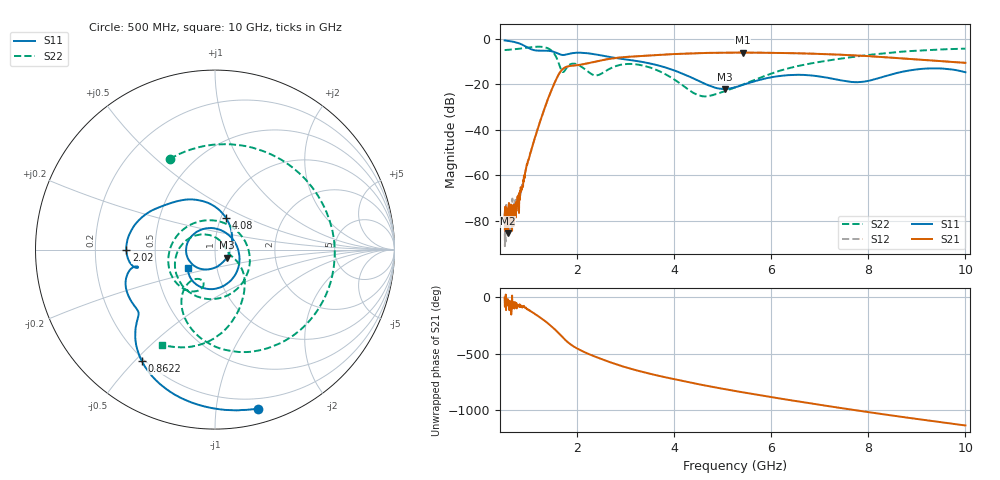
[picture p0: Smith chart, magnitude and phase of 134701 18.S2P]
!  2-Port S-parameters saved by WinCal
! VAR MeasName=S-Parameters (CALIBRATED_DATA) read from VNA (N5242A)
! VAR MeasDate=2013-7-3 16:31:00
! VAR NAME=134701 18
! VAR FILENAME=134701 18.S2P
! VAR DATE=2013-7-3 16:31:00
! VAR PHYS_PORTS=1,2
# Hz S MA R 50
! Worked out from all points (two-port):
!   1601 points, 500 MHz to 10 GHz, reference 50 ohm
!   highest |S21| = -6.09 dB at 5.41 GHz (marker M1); lowest = -85.5 dB at 565.3 MHz (marker M2)
!   |S21| within 3 dB of the highest: 2.592 GHz to 8.999 GHz (6.407 GHz wide, 111 % of centre)
!   lowest |S11| = -22.1 dB at 5.036 GHz (marker M3), VSWR 1.17, Z = 56.6 - j5.16 ohm
!   |S11| at or under -10 dB: 3.286 GHz to end of sweep
!   |S22| runs from -25.4 to -3.5 dB; largest |S21 - S12| = 0.0022
!   S11 on the Smith chart (normalised r, x): 500 MHz: 0.12, -1.30; 862.2 MHz: 0.19, -0.52; 2.02 GHz: 0.34, -0.00; 4.08 GHz: 1.06, +0.39; 10 GHz: 0.72, -0.15
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5e8  0.9175 -74.8  0.0001227 -4.8  0.000148 -52.6  0.5644 116.6
5.653125e8  0.8996 -83.9  5.304e-05 -55.7  0.0001652 -62.7  0.5707 107.3
7.196875e8  0.8404 -105.2  0.0002006 -45.6  0.0002437 -47.8  0.5909 83.7
8.621875e8  0.7426 -123.3  0.0005362 -92.3  0.000619 -88.5  0.6158 59.3
1.165e9  0.5499 -141.1  0.009124 -161.0  0.009129 -160.3  0.6681 -4.1
1.4025e9  0.5442 -154.6  0.05017 124.5  0.05006 124.3  0.6095 -67.8
1.550938e9  0.4982 -165.4  0.1206 68.7  0.1204 68.5  0.4198 -113.2
1.699375e9  0.4395 -167.2  0.216 2.6  0.2155 2.5  0.1853 -116.9
2.02e9  0.4942 -179.9  0.2641 -100.7  0.2636 -100.8  0.2658 -168.3
2.085312e9  0.4931 175.8  0.271 -115.0  0.2704 -115.1  0.2422 172.8
2.607812e9  0.4084 147.0  0.3537 153.6  0.3535 153.5  0.2023 -16.1
3.005625e9  0.35 131.0  0.3978 97.4  0.3971 97.4  0.2781 -97.7
3.670625e9  0.2585 96.8  0.4421 23.9  0.441 24.0  0.1978 177.2
4.080312e9  0.1866 70.7  0.4653 -14.8  0.465 -14.7  0.1106 130.0
4.567188e9  0.11 29.3  0.4849 -57.0  0.4852 -57.0  0.05473 49.2
5.03625e9  0.07874 -35.1  0.4941 -94.8  0.4951 -94.8  0.07003 -8.4
5.25e9  0.08539 -65.8  0.4953 -111.2  0.496 -111.3  0.08485 -17.6
5.410312e9  0.09691 -84.8  0.4959 -123.2  0.4958 -123.2  0.09834 -21.4
6.110938e9  0.1486 -144.5  0.4887 -173.5  0.4891 -173.6  0.188 -36.5
6.835312e9  0.1554 160.2  0.4703 137.1  0.4702 137.0  0.2895 -56.2
8.420625e9  0.1583 -32.5  0.3887 35.6  0.3877 35.5  0.4898 -89.8
1e10  0.1836 -145.7  0.2958 -56.5  0.295 -56.8  0.6061 -118.9
